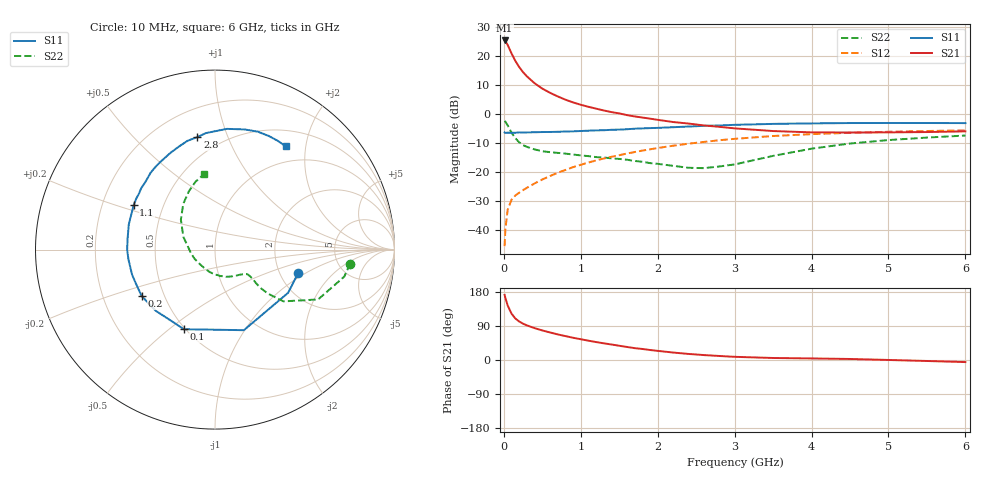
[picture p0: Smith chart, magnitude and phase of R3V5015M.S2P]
! SIEMENS Small Signal Semiconductors
! BFR181
! Si NPN RF Bipolar Junction Transistor in SOT23
! VCE = 0.5 V  IC = 15 mA
! Common Emitter S-Parameters:  May  1996
# GHz  S  MA  R  50
!  f  S11  S21  S12  S22
! GHz  MAG  ANG  MAG  ANG  MAG  ANG  MAG  ANG
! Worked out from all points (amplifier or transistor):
!   36 points, 10 MHz to 6 GHz, reference 50 ohm
!   highest |S21| = 25.3 dB at 10 MHz (marker M1)
!   |S21| within 3 dB of that: start of sweep to 74.81 MHz
!   unconditionally stable (mu >= 1): start of sweep to 19.61 MHz; 145 MHz to end of sweep
!   at 250 MHz: K = 1.37, MAG = 16.7 dB, |S12| = -26.2 dB
!   at 1.4 GHz: K = 1.77, MAG = 2.6 dB, |S12| = -14.7 dB
!   at 6 GHz: K = 1.21, MAG = -2.9 dB, |S12| = -5.6 dB
!   S11 on the Smith chart (normalised r, x): 10 MHz: 2.51, -0.87; 100 MHz: 0.49, -0.56; 200 MHz: 0.37, -0.25; 1.1 GHz: 0.34, +0.23; 2.8 GHz: 0.37, +0.78; 6 GHz: 0.74, +1.65
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0.01  0.4812 -16.0  18.48 171.8  0.0053 75.8  0.7567 -5.9
0.02  0.4732 -30.6  17.93 163.9  0.0104 74.2  0.736 -11.8
0.05  0.4769 -70.3  15.46 143.7  0.0225 62.2  0.6381 -25.8
0.1  0.4761 -111.3  11.04 122.3  0.0336 52.2  0.4782 -37.1
0.15  0.4746 -134.2  8.189 109.5  0.0396 49.6  0.3823 -39.8
0.2  0.4836 -147.7  6.429 101.5  0.0442 49.9  0.3255 -40.1
0.25  0.4795 -156.1  5.252 95.8  0.0489 51.8  0.2915 -39.1
0.3  0.4827 -163.1  4.447 91.3  0.0537 53.7  0.2718 -38.1
0.4  0.4853 -173.4  3.387 84.1  0.0638 57.0  0.2458 -37.2
0.5  0.4894 -179.8  2.739 78.0  0.0745 59.4  0.2288 -37.2
0.6  0.4906 173.6  2.319 72.7  0.0855 60.8  0.2204 -38.1
0.8  0.5001 163.9  1.768 63.1  0.1089 62.3  0.2082 -41.2
0.9  0.503 159.9  1.583 58.7  0.1216 62.7  0.2005 -43.9
1.1  0.5164 151.3  1.33 51.0  0.1461 62.2  0.1882 -50.2
1.3  0.5259 143.7  1.15 44.0  0.1712 60.9  0.1782 -56.4
1.6  0.547 133.4  0.958 34.4  0.2086 58.3  0.1633 -67.9
2.2  0.5927 115.0  0.728 19.7  0.2844 50.8  0.1282 -103.9
2.8  0.6343 98.9  0.602 10.6  0.3536 41.7  0.1249 -156.0
3.5  0.6759 84.4  0.509 5.3  0.4181 30.7  0.1901 158.0
4.5  0.699 70.0  0.48 2.7  0.4749 16.2  0.3105 124.7
5.5  0.6997 60.0  0.489 -2.6  0.51 4.3  0.393 106.1
6  0.6974 55.6  0.503 -5.5  0.5219 -1.6  0.4259 98.1
